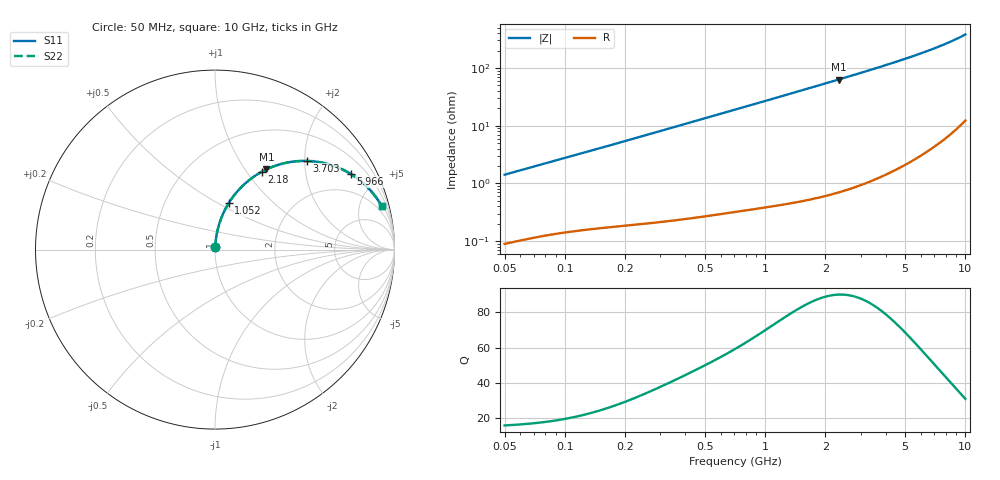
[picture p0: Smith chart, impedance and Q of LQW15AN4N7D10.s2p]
!Murata Part Number: LQW15AN4N7D10
!These Parameters are Measured in Series Mode Connection
!  o--[Z]--o
!Port1  Port2
!  o-------o
!Freq. Start=50[MHz] Stop=10[GHz], 401[Steps]
# Hz S RI R 50
!Freq.(Hz)	S 11(Real)	S 11(Imag)	S 21(Real)	S 21(Imag)	S 12(Real)	S 12(Imag)	S 22(Real)	S 22(Imag)
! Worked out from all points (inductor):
!   401 points, 50 MHz to 10 GHz, reference 50 ohm
!   read as one part in series: L = 4.46 nH near 51.34 MHz
!   highest Q = 90.1 at 2.329 GHz (marker M1), where L = 4.31 nH
!   S11 on the Smith chart (normalised r, x): 50 MHz: 1.00, +0.03; 1.052 GHz: 1.01, +0.56; 2.18 GHz: 1.01, +1.18; 3.703 GHz: 1.03, +2.05; 5.966 GHz: 1.06, +3.55; 10 GHz: 1.25, +7.59
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5e7  0.0011 0.0141  0.9989 -0.0141  0.9989 -0.0141  0.0011 0.0141
1.214486e8  0.00265 0.0331  0.9974 -0.0331  0.9974 -0.0331  0.00265 0.0331
1.956524e8  0.00463 0.0527  0.9954 -0.0527  0.9954 -0.0527  0.00463 0.0527
2.949953e8  0.00838 0.0787  0.9916 -0.0787  0.9916 -0.0787  0.00838 0.0787
4.689809e8  0.0181 0.1234  0.9819 -0.1234  0.9819 -0.1234  0.0181 0.1234
7.071068e8  0.0375 0.1818  0.9625 -0.1818  0.9625 -0.1818  0.0375 0.1818
1.052113e9  0.0766 0.2591  0.9234 -0.2591  0.9234 -0.2591  0.0766 0.2591
1.353197e9  0.1193 0.318  0.8807 -0.318  0.8807 -0.318  0.1193 0.318
1.717543e9  0.1785 0.3772  0.8215 -0.3772  0.8215 -0.3772  0.1785 0.3772
2.179987e9  0.2597 0.433  0.7403 -0.433  0.7403 -0.433  0.2597 0.433
2.329253e9  0.2864 0.4466  0.7136 -0.4466  0.7136 -0.4466  0.2864 0.4466
2.956399e9  0.3961 0.4834  0.6039 -0.4834  0.6039 -0.4834  0.3961 0.4834
3.330706e9  0.4571 0.4923  0.5429 -0.4923  0.5429 -0.4923  0.4571 0.4923
3.703027e9  0.5133 0.4938  0.4867 -0.4938  0.4867 -0.4938  0.5133 0.4938
4.171863e9  0.5772 0.4876  0.4228 -0.4876  0.4228 -0.4876  0.5772 0.4876
4.955797e9  0.6671 0.4641  0.3329 -0.4641  0.3329 -0.4641  0.6671 0.4641
5.965537e9  0.7556 0.4214  0.2444 -0.4214  0.2444 -0.4214  0.7556 0.4214
6.810442e9  0.811 0.382  0.189 -0.382  0.189 -0.382  0.811 0.382
7.775012e9  0.8589 0.3371  0.1411 -0.3371  0.1411 -0.3371  0.8589 0.3371
8.994549e9  0.9025 0.2833  0.0975 -0.2833  0.0975 -0.2833  0.9025 0.2833
9.738562e9  0.9223 0.2527  0.0777 -0.2527  0.0777 -0.2527  0.9223 0.2527
1e10  0.9283 0.2424  0.0717 -0.2424  0.0717 -0.2424  0.9283 0.2424
